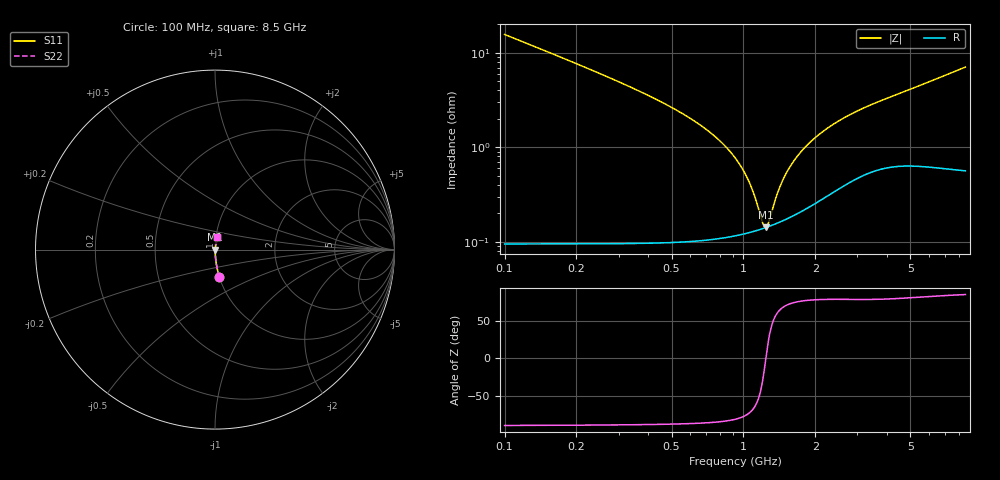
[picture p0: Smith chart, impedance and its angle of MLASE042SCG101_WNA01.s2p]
! MLASE042SCG101_WNA01  S-PARAMETER MODEL  ( General Type )
! Model Generated by TAIYO YUDEN Corporation (http://www.ty-top.com)
! Version 4.0
! TAIYO YUDEN Control No. 180301
! Copyright(c) 2013 TAIYO YUDEN CO.,LTD. All Rights Reserved.
! Product Description (link to TY-COMPAS)
! https://ds.yuden.co.jp/TYCOMPAS/or/detail?pn=MLASE042SCG101JWNA01&u=M
! Products Name : Multilayer Ceramic Capacitors
! Characteristics :
!  Capacitance : 100 pF , Rated Voltage : 16V , TCC : CG / C0G
!  Case Size : 0.4 x 0.2 / 0.016 x 0.008 [mm/inch] , Thickness : 0.2 / 0.008 [mm/inch]
!  (Conditions: Temperature = 25 degC , DC Bias Current/Voltage = 0A / 0V)
! External Node Assignments :
!  1  o---| |---o  2
! GND o---------o GND
! Frequency Range : 100MHz  -  8500MHz  [ 401 STEP ]
# MHz S RI R 50
! Freq[MHz].  S11 Real  S11 Imag  S21 Real  S21 Imag  S12 Real  S12 Imag  S22 Real  S22 Imag
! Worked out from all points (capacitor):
!   401 points, 100 MHz to 8.5 GHz, reference 50 ohm
!   read as one part in series: C = 101 pF near 102.2 MHz
!   lowest |Z| = 142 mohm at 1.244 GHz (marker M1)
!   series resonance near 1.241 GHz, so ESL is about 160 pH
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100  0.0248 -0.1526  0.9752 0.1526  0.9752 0.1526  0.0248 -0.1526
141.101  0.0129 -0.1088  0.9871 0.1088  0.9871 0.1088  0.0129 -0.1088
186.2596  0.00773 -0.082  0.9923 0.082  0.9923 0.082  0.00773 -0.082
310.4573  0.00321 -0.0474  0.9968 0.0474  0.9968 0.0474  0.00321 -0.0474
447.8978  0.00191 -0.0306  0.9981 0.0306  0.9981 0.0306  0.00191 -0.0306
806.9133  0.00121 -0.0113  0.9988 0.0113  0.9988 0.0113  0.00121 -0.0113
963.8371  0.00122 -0.00649  0.9988 0.00649  0.9988 0.00649  0.00122 -0.00649
1077.058  0.00128 -0.00361  0.9987 0.00361  0.9987 0.00361  0.00128 -0.00361
1203.579  0.00138 -0.000778  0.9986 0.000778  0.9986 0.000778  0.00138 -0.000778
1244.358  0.00142 6.75e-05  0.9986 -6.75e-05  0.9986 -6.75e-05  0.00142 6.75e-05
1272.308  0.00144 0.000631  0.9986 -0.000631  0.9986 -0.000631  0.00144 0.000631
1406.061  0.0016 0.00317  0.9984 -0.00317  0.9984 -0.00317  0.0016 0.00317
1502.954  0.00174 0.00487  0.9983 -0.00487  0.9983 -0.00487  0.00174 0.00487
1606.523  0.00191 0.00659  0.9981 -0.00659  0.9981 -0.00659  0.00191 0.00659
1717.229  0.0021 0.00832  0.9979 -0.00832  0.9979 -0.00832  0.0021 0.00832
2006.124  0.0027 0.0124  0.9973 -0.0124  0.9973 -0.0124  0.0027 0.0124
2396.263  0.00366 0.0173  0.9963 -0.0173  0.9963 -0.0173  0.00366 0.0173
2926.566  0.00504 0.0229  0.995 -0.0229  0.995 -0.0229  0.00504 0.0229
4317.005  0.00741 0.0347  0.9926 -0.0347  0.9926 -0.0347  0.00741 0.0347
5762.285  0.00835 0.0464  0.9916 -0.0464  0.9916 -0.0464  0.00835 0.0464
7116.102  0.00923 0.0577  0.9908 -0.0577  0.9908 -0.0577  0.00923 0.0577
8500  0.0105 0.0694  0.9895 -0.0694  0.9895 -0.0694  0.0105 0.0694
